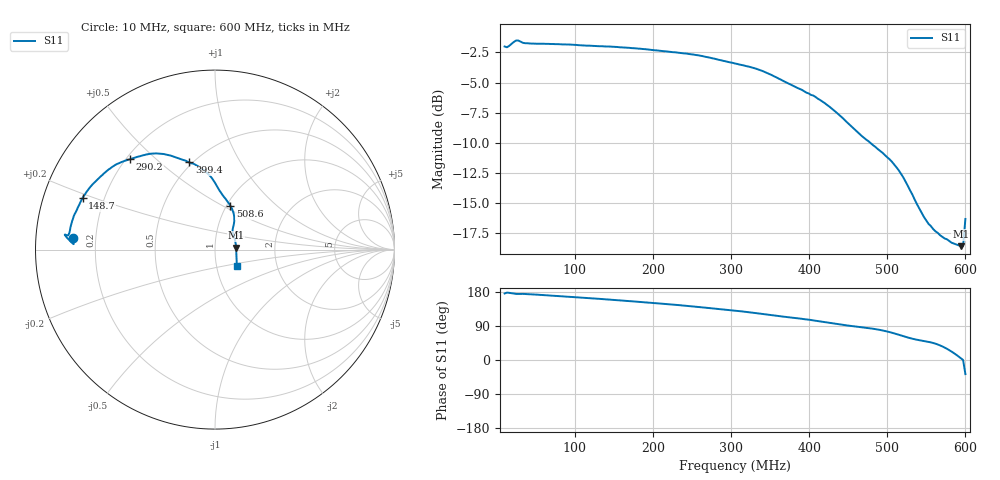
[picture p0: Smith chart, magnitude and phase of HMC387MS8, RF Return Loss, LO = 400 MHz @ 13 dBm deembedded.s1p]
!Hittite Microwave Corporation
!12 Elizabeth Drive
!Chelmsford, MA 01824
!Tel: 978-250-3343
!Fax: 978-250-3373
!Device: HMC387MS8, 450-500 MHz, GaAs MMIC High IP3 Mixer in 8-lead plastic SMT package
!Misc: RF Return Loss, LO = 400 MHz @ 13 dBm, Room
# MHZ S MA R 50
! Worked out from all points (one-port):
!   201 points, 10 MHz to 600 MHz, reference 50 ohm
!   lowest |S11| = -18.6 dB at 594.1 MHz (marker M1), VSWR 1.27, Z = 63.3 + j1.27 ohm
!   |S11| at or under -10 dB: 478.4 MHz to end of sweep
!   S11 on the Smith chart (normalised r, x): 10 MHz: 0.12, +0.04; 148.7 MHz: 0.12, +0.19; 290.2 MHz: 0.21, +0.41; 399.4 MHz: 0.48, +0.63; 508.6 MHz: 1.04, +0.54; 600 MHz: 1.25, -0.24
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10  0.794 175.5
12.95  0.788 177.8
24.75  0.841 174.4
33.6  0.822 174.5
83.75  0.81 168.0
148.65  0.792 158.7
157.5  0.788 157.3
189.95  0.774 152.2
231.25  0.749 145.2
260.75  0.727 139.3
290.25  0.692 133.3
305  0.675 130.2
340.4  0.628 121.4
358.1  0.591 116.6
378.75  0.547 111.7
399.4  0.507 106.4
425.95  0.447 98.0
452.5  0.374 90.2
493.8  0.288 78.0
508.55  0.258 70.5
517.4  0.236 64.9
526.25  0.21 59.4
543.95  0.162 51.3
552.8  0.146 48.0
573.45  0.127 32.8
594.1  0.118 4.8
597.05  0.118 -0.0
600  0.153 -37.2
